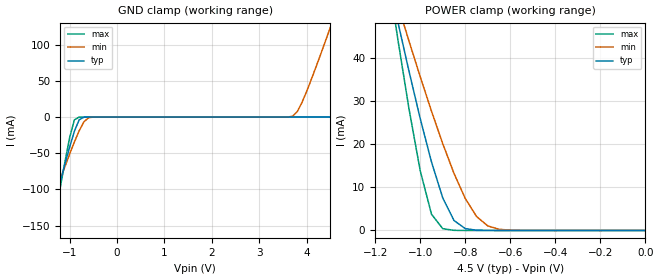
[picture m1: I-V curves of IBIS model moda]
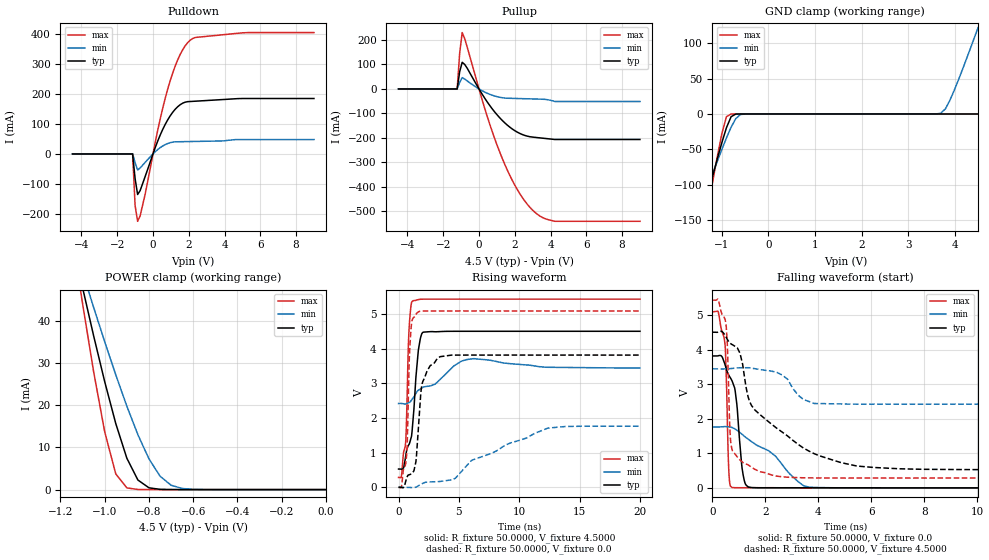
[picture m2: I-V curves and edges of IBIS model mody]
| IBIS (I/O, Buffer, Information, Specification) Model, officially
| electronic behavioral standard for Buffer structures of digital pins.
[IBIS ver]  4.0
[File name] 54ac04_4v5_rev1.ibs
[File Rev] 1.0
[Date]  30 June 2009
[Source] CAD & Design Solution (Catania) - STMicroelectronics
[Notes]
  (Note1) This IBIS model is the model of the product with package
   (Flat14 package elements);
  (Note2) This IBIS model is extracted with nominal 4.5V power supply
   (min:3.0V, typ:4.5V, max:5.5V);
  (Note3) This model has few Warnings about the non-monotonicity
   of I-V curves, but they are not indicative of problems
   inside the model;
[Copyright] (c) 2009 STMicroelectronics
|   Component 54AC04
[Component] 54AC04
[Manufacturer] STMicroelectronics
[Package]
| variable   typ   min   max
R_pkg   0.0   0.0   0.0
L_pkg   0.0H   0.0H   0.0H
C_pkg   0.0F   0.0F   0.0F
[Pin]  signal_name   model_name   R_pin   L_pin   C_pin
1   A0   moda   141.0m   4.31nH   1.01pF
2   O0   mody   108.1m   3.05nH   1.04pF
3   A1   moda   90.5m   2.36nH   0.8pF
4   O1   mody   79.7m   1.96nH   0.8pF
5   A2   moda   86.2m   2.16nH   0.8pF
6   O2   mody   101.7m   2.85nH   1.04pF
7   GND   GND   111.0m   3.51nH   1.01pF
8   O5   mody   141.0m   4.31nH   1.01pF
9   A5   moda   112.4m   3.25nH   1.04pF
10   O4   mody   90.5m   2.36nH   0.8pF
11   A4   moda   81.9m   2.06nH   0.8pF
12   O3   mody   84.0m   2.16nH   0.8pF
13   A3   moda   101.7m   2.85nH   1.04pF
14   VCC   POWER   111.0m   3.51nH   1.01pF
| Models and submodels in the file (2): moda (Input), mody (I/O)
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|   Model moda
[Model]  moda
Model_type Input
Vinl =   1.35V
Vinh =   3.15V
C_comp   0.532pF   NA   NA
[Temperature Range]   25.0000   0.1250k   -55.0000
[Voltage Range]   4.5000V   3.0000V   5.5000V
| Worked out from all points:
|   GND clamp passes 1 mA (typ) near -0.72 V on its own axis
|   POWER clamp passes 1 mA (typ) near -0.82 V on its own axis
[GND_clamp]
|Voltage   I(typ)   I(min)   I(max)
-4.5V     -962.5mA   -710.6mA   -1.378A
-1.7V     -218.5mA   -178.3mA   -287.1mA
-1.6V     -192.5mA   -159.7mA   -248.8mA
-1.5V     -166.5mA   -141.2mA   -210.6mA
-1.4V     -140.8mA   -122.8mA   -172.7mA
-1V       -41.47mA   -51.24mA   -28.54mA
-900mV    -19.68mA   -34.52mA   -3.902mA
-800mV    -3.919mA   -19.11mA   -32.25uA
-500mV    -58.62nA   -53.84uA   -16.8pA
3.7V      5.8pA      1.051mA    3.8pA
3.9V      6.6pA      20.13mA    4.6pA
4.5V      9.001pA    124.1mA    7pA
[POWER_clamp]
|Voltage   I(typ)   I(min)   I(max)
-4.5V     943.9mA    692.8mA    1.358A
-1.15V    60.51mA    61.11mA    61.84mA
-1.1V     48.57mA    52.46mA    44.58mA
-1.05V    36.98mA    43.96mA    28.26mA
-1V       25.96mA    35.67mA    13.85mA
-950mV    15.89mA    27.69mA    3.78mA
-900mV    7.563mA    20.13mA    416.9uA
-850mV    2.308mA    13.24mA    30.74uA
-750mV    65.13uA    3.242mA    151.1nA
-700mV    9.377uA    1.051mA    10.58nA
-600mV    191.5nA    66.07uA    65.13pA
0V        4.5pA      41.65pA    3.7pA
|   Model mody
[Model]   mody
Model_type I/O
Polarity   Inverting
Vinl   =   1.35V
Vinh   =   3.15V
Vmeas  =   2.25V
Cref   =   50pf
Rref   =   500
C_comp   3.355pF   NA   NA
[Temperature Range]   25.0000   0.1250k   -55.0000
[Voltage Range]   4.5000V   3.0000V   5.5000V
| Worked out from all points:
|   slope of the pulldown table from 0 to 0.675 V, typ, clamps not added: 6.92 ohm
|   slope of the pullup table from 0 to 0.675 V, typ, clamps not added: 8.98 ohm
|   GND clamp passes 1 mA (typ) near -0.72 V on its own axis
|   POWER clamp passes 1 mA (typ) near -0.82 V on its own axis
|   rising waveform, R_fixture 50.0000, V_fixture 4.5000: 20-80 % time 621ps typ, 2.52ns min, 256ps max; typ from 0.527 V to 4.5 V
|   rising waveform, R_fixture 50.0000, V_fixture 0.0: 20-80 % time 567ps typ, 5.55ns min, 257ps max; typ from 0 V to 3.81 V
|   falling waveform, R_fixture 50.0000, V_fixture 0.0: 20-80 % time 332ps typ, 1.65ns min, 110ps max; typ from 3.81 V to 0 V
|   falling waveform, R_fixture 50.0000, V_fixture 4.5000: 20-80 % time 2.03ns typ, 649ps min, 149ps max; typ from 4.5 V to 0.527 V
[Pulldown]
|Voltage   I(typ)   I(min)   I(max)
-4.5V     0A         0A         0A
-1.14V    0A         0A         0A
-1V       -82.5mA    -29.34mA   -172.5mA
-860mV    -135.4mA   -53.46mA   -224.7mA
-440mV    -75.65mA   -28.24mA   -134.8mA
260mV     42.23mA    14.38mA    77.67mA
820mV     113.3mA    34.67mA    215.6mA
1.38V     157.3mA    40.54mA    313.4mA
1.94V     174.3mA    41.15mA    371.1mA
2.36V     175.8mA    41.61mA    388.1mA
5.02V     184.8mA    47.96mA    403.9mA
9V        184.8mA    47.96mA    404.7mA
[Pullup]
|Voltage   I(typ)   I(min)   I(max)
-4.5V     0A         0A         0A
-1.22V    0A         0A         0A
-1.08V    70.6mA     26.5mA     146.9mA
-940mV    108.9mA    46.2mA     230.5mA
-800mV    100.1mA    40.39mA    205.9mA
460mV     -53.18mA   -17.69mA   -112.6mA
1.16V     -118.1mA   -34.17mA   -258.5mA
2V        -170.6mA   -38.91mA   -393.2mA
2.84V     -195.4mA   -40.6mA    -483.8mA
3.54V     -201.3mA   -42.06mA   -525.6mA
4.24V     -206.8mA   -51.45mA   -541.4mA
9V        -206.8mA   -51.45mA   -541.4mA
[GND_clamp]
|Voltage   I(typ)   I(min)   I(max)
-4.5V     -947.8mA   -697.3mA   -1.362A
-1.7V     -215.2mA   -175mA     -283.7mA
-1.6V     -189.5mA   -156.7mA   -245.8mA
-1.5V     -164mA     -138.6mA   -208.1mA
-1.4V     -138.6mA   -120.5mA   -170.6mA
-1V       -40.81mA   -50.28mA   -28.18mA
-900mV    -19.37mA   -33.88mA   -3.841mA
-800mV    -3.851mA   -18.75mA   -31.64uA
-500mV    -57.51nA   -52.83uA   -10.23pA
3.7V      2.9pA      1.031mA    1.9pA
3.9V      3.3pA      19.76mA    2.3pA
4.5V      4.5pA      121.8mA    3.5pA
[POWER_clamp]
|Voltage   I(typ)   I(min)   I(max)
-4.5V     929.4mA    679.8mA    1.342A
-1.15V    59.57mA    59.97mA    61.08mA
-1.1V     47.81mA    51.47mA    44.01mA
-1.05V    36.4mA     43.14mA    27.9mA
-1V       25.55mA    35.01mA    13.66mA
-950mV    15.63mA    27.17mA    3.721mA
-900mV    7.436mA    19.76mA    409.3uA
-850mV    2.267mA    13mA       30.16uA
-750mV    63.91uA    3.182mA    148.2nA
-700mV    9.201uA    1.031mA    10.38nA
-600mV    187.9nA    64.84uA    57.46pA
0V        4.5pA      41.65pA    5.5pA
[Ramp]
| variable   typ   min   max
dV/dt_r  2.2886/0.7438n   1.0570/5.5380n   3.0522/0.5052n
dV/dt_f  2.3840/2.1085n   1.1659/16.1241n   3.0890/0.3656n
R_load = 50.0000
[Rising Waveform]
R_fixture= 50.0000
V_fixture= 4.5000
|time   V(typ)   V(min)   V(max)
0s        526.6mV    2.416V     283.7mV
220ps     524.7mV    2.419V     278.5mV
600ps     911.7mV    2.406V     1.333V
840ps     1.221V     2.439V     4.329V
1ns       1.377V     2.477V     5.135V
1.16ns    1.774V     2.555V     5.371V
1.64ns    3.949V     2.799V     5.414V
2ns       4.467V     2.879V     5.427V
6.24ns    4.5V       3.712V     5.428V
20ns      4.5V       3.441V     5.428V
[Rising Waveform]
R_fixture= 50.0000
V_fixture= 0.0
|time   V(typ)   V(min)   V(max)
0s        0V         0V         0V
680ps     280.7mV    -1.107mV   982.4mV
880ps     360.6mV    -4.191mV   3.6V
1.08ns    387.5mV    -7.254mV   4.732V
1.44ns    738.8mV    4.573mV    4.982V
1.6ns     1.478V     33.58mV    5.05V
1.96ns    2.992V     106.6mV    5.084V
3.44ns    3.768V     167.5mV    5.087V
12.36ns   3.813V     1.706V     5.087V
20ns      3.814V     1.762V     5.087V
[Falling Waveform]
R_fixture= 50.0000
V_fixture= 0.0
|time   V(typ)   V(min)   V(max)
0s        3.814V     1.762V     5.087V
220ps     3.818V     1.76V      5.084V
480ps     3.55V      1.772V     4.121V
620ps     3.254V     1.763V     457.7mV
740ps     3.096V     1.745V     11.32mV
920ps     2.425V     1.667V     4.311mV
1.12ns    566.1mV    1.547V     3.736mV
1.36ns    24.8mV     1.402V     5.746mV
3.64ns    2.352mV    22.95mV    612.6uV
20ns      16.21uV    667uV      3.437uV
[Falling Waveform]
R_fixture= 50.0000
V_fixture= 4.5000
|time   V(typ)   V(min)   V(max)
0s        4.5V       3.44V      5.428V
520ps     4.351V     3.441V     4.672V
660ps     4.188V     3.447V     1.665V
740ps     4.144V     3.453V     1.107V
1.04ns    3.894V     3.472V     807.3mV
1.42ns    2.472V     3.469V     627.9mV
1.8ns     2.116V     3.42V      467.8mV
3.84ns    990.2mV    2.439V     287.7mV
5.46ns    630.9mV    2.42V      283.8mV
20ns      526.5mV    2.42V      283.5mV
